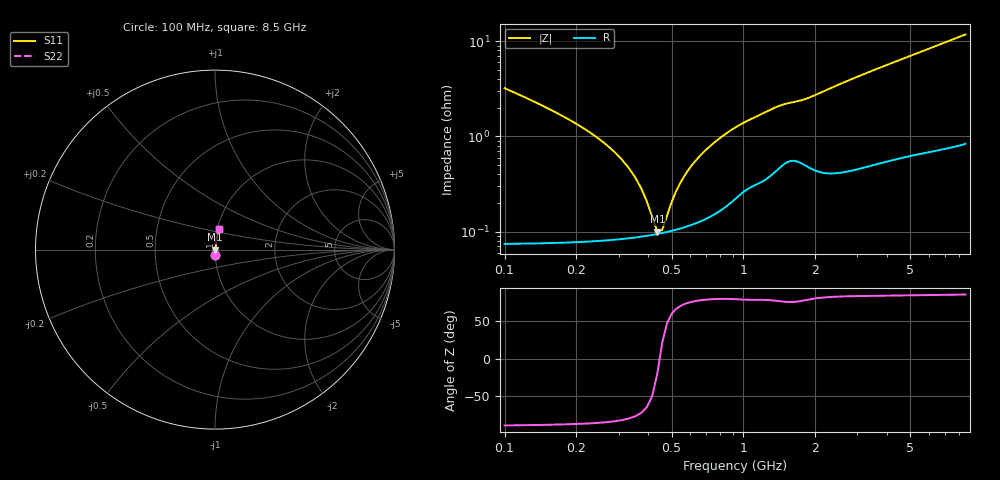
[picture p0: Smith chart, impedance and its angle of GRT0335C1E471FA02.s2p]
!Murata Part Number: GRT0335C1E471FA02
!These Parameters are Measured in Series Mode Connection
!Data Generated on Jun 19, 2026
!  o--ll--o
!Port1  Port2
!  o------o
!Operation Temp=25[degC], DC Bias Voltage=0[V]
!Freq. Start=100[MHz] Stop=9[GHz] 401[Steps]
# Hz S RI R 50
!Freq.(Hz) S11(Real) S11(Imag) S21(Real) S21(Imag) S12(Real) S12(Imag) S22(Real) S22(Imag)
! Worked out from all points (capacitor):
!   401 points, 100 MHz to 8.5 GHz, reference 50 ohm
!   read as one part in series: C = 470 pF near 142 MHz
!   lowest |Z| = 100 mohm at 436 MHz (marker M1)
!   series resonance near 445.7 MHz, so ESL is about 270 pH
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1e8  0.00178 -0.0321  0.9982 0.0321  0.9982 0.0321  0.00178 -0.0321
1.42e8  0.00121 -0.0214  0.9988 0.0214  0.9988 0.0214  0.00121 -0.0214
3.1e8  0.000869 -0.00564  0.9991 0.00564  0.9991 0.00564  0.000869 -0.00564
3.52e8  0.000882 -0.00362  0.9991 0.00362  0.9991 0.00362  0.000882 -0.00362
4.15e8  0.000926 -0.00108  0.9991 0.00108  0.9991 0.00108  0.000926 -0.00108
4.36e8  0.000946 -0.000332  0.9991 0.000332  0.9991 0.000332  0.000946 -0.000332
4.57e8  0.000969 0.000385  0.999 -0.000385  0.999 -0.000385  0.000969 0.000385
4.78e8  0.000994 0.00107  0.999 -0.00107  0.999 -0.00107  0.000994 0.00107
5.41e8  0.00108 0.00298  0.9989 -0.00298  0.9989 -0.00298  0.00108 0.00298
5.62e8  0.00112 0.00358  0.9989 -0.00358  0.9989 -0.00358  0.00112 0.00358
6.04e8  0.0012 0.00472  0.9988 -0.00472  0.9988 -0.00472  0.0012 0.00472
6.88e8  0.00139 0.00687  0.9986 -0.00687  0.9986 -0.00687  0.00139 0.00687
7.72e8  0.00165 0.00887  0.9984 -0.00887  0.9984 -0.00887  0.00165 0.00887
8.98e8  0.00221 0.0116  0.9978 -0.0116  0.9978 -0.0116  0.00221 0.0116
1.024e9  0.00292 0.014  0.9971 -0.014  0.9971 -0.014  0.00292 0.014
1.297e9  0.00418 0.0186  0.9958 -0.0186  0.9958 -0.0186  0.00418 0.0186
1.507e9  0.0057 0.0212  0.9943 -0.0212  0.9943 -0.0212  0.0057 0.0212
2.914e9  0.00607 0.0405  0.9939 -0.0405  0.9939 -0.0405  0.00607 0.0405
4.3e9  0.00926 0.0595  0.9907 -0.0595  0.9907 -0.0595  0.00926 0.0595
5.707e9  0.0128 0.078  0.9872 -0.078  0.9872 -0.078  0.0128 0.078
7.114e9  0.0168 0.0962  0.9832 -0.0962  0.9832 -0.0962  0.0168 0.0962
8.5e9  0.0216 0.114  0.9784 -0.114  0.9784 -0.114  0.0216 0.114
